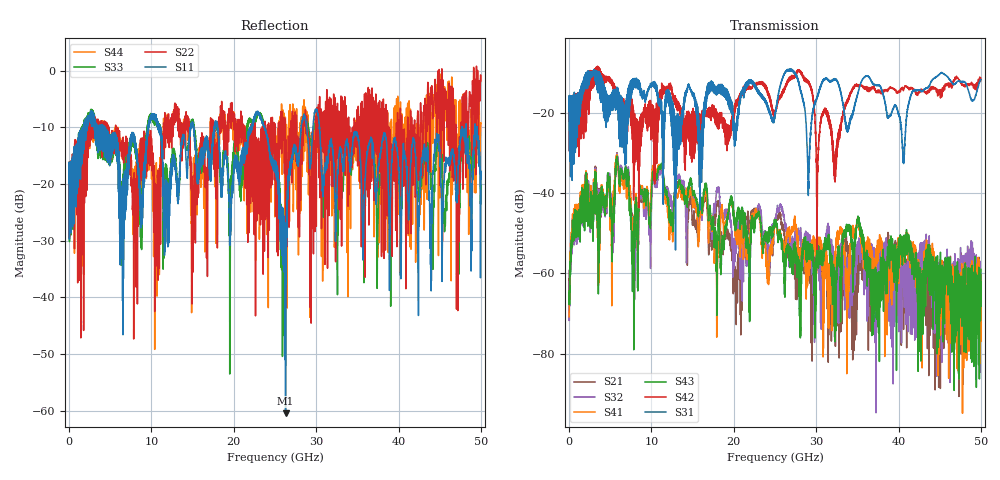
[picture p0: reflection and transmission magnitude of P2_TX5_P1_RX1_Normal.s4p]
!Keysight Technologies,N5225B,MY57041031,A.13.20.10
!Date: Friday, May 31, 2019 11:14:56
!Correction: S11(Full 4 Port(1,2,3,4))
!S12(Full 4 Port(1,2,3,4))
!S13(Full 4 Port(1,2,3,4))
!S14(Full 4 Port(1,2,3,4))
!S21(Full 4 Port(1,2,3,4))
!S22(Full 4 Port(1,2,3,4))
!S23(Full 4 Port(1,2,3,4))
!S24(Full 4 Port(1,2,3,4))
!S31(Full 4 Port(1,2,3,4))
!S32(Full 4 Port(1,2,3,4))
!S33(Full 4 Port(1,2,3,4))
!S34(Full 4 Port(1,2,3,4))
!S41(Full 4 Port(1,2,3,4))
!S42(Full 4 Port(1,2,3,4))
!S43(Full 4 Port(1,2,3,4))
!S44(Full 4 Port(1,2,3,4))
!S4P File: Measurements: <S11,S12,S13,S14>,
!<S21,S22,S23,S24>,
!<S31,S32,S33,S34>,
!<S41,S42,S43,S44>:
# Hz S  dB  R 50.0
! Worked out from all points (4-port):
!   5000 points, 10 MHz to 50 GHz, reference 50 ohm
!   strongest paths, dB at 10 MHz, 12.51 GHz, 25.01 GHz, 37.51 GHz, 50 GHz:
!     S31: -19.5, -17.8, -20.9, -13.1, -11.7
!     S42: -19.5, -14.6, -19.9, -14.7, -11.4
!     S43: -66.3, -45.9, -47.5, -61.9, -59.0
!     S41: -70.7, -47.6, -47.5, -53.5, -70.5
!     S32: -62.2, -43.0, -47.0, -56.6, -62.7
!     S21: -59.3, -42.7, -47.0, -55.6, -67.3
!   lowest |S11| = -60.5 dB at 26.29 GHz (marker M1), VSWR 1.00, Z = 50.1 - j0.0668 ohm
!   |S11| at or under -10 dB: 4.282 GHz to 9.568 GHz (5.286 GHz wide, 76.3 % of centre); 23.74 GHz to 28.18 GHz (4.44 GHz wide, 17.1 % of centre); 30.39 GHz to 47.71 GHz (17.32 GHz wide, 44.3 % of centre)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
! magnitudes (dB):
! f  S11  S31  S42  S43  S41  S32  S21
! 10 MHz  -19.8  -19.5  -19.5  -66.3  -70.7  -62.2  -59.3
! 5.78 GHz  -12.1  -14.9  -14.5  -31.2  -30.7  -30.9  -30.5
! 20.19 GHz  -16.0  -27.1  -17.6  -49.3  -50.7  -52.6  -64.3
! 22.93 GHz  -7.2  -14.9  -12.7  -45.1  -45.1  -43.3  -44.0
! 26.29 GHz  -60.5  -9.7  -13.7  -58.3  -54.4  -48.6  -52.4
! 30.01 GHz  -6.8  -16.7  -32.4  -56.2  -57.9  -57.5  -54.9
! 50 GHz  -19.1  -11.7  -11.4  -59.0  -70.5  -62.7  -67.3
